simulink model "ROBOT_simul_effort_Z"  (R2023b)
settings: Solver=VariableStepAuto  StartTime=0.0  StopTime=5  RelTol=1e-3
undefined symbols (not defined in the file): deg, kg, m, manette1_Defaut_sldprt, manette2_Defaut_sldprt, mm, N, rad, s, STL, X, Y, Z
libraries: sm_lib x463, fl_lib x45, nesl_utility x27, simulink x2
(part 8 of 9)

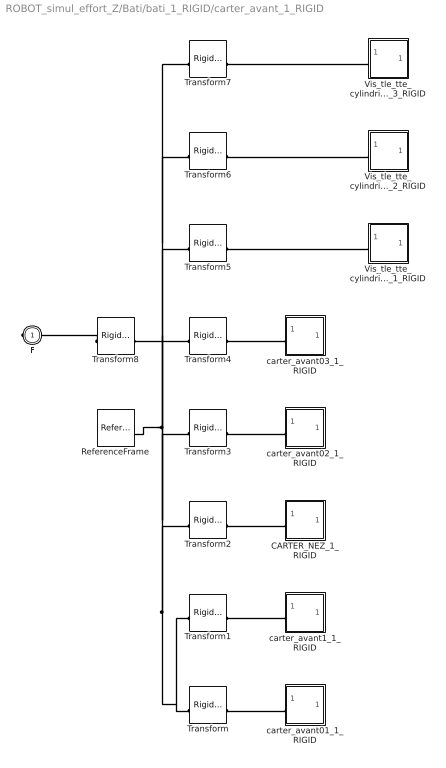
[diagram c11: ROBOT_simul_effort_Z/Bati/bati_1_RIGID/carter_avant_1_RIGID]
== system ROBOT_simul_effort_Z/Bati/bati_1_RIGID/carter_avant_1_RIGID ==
  CARTER_NEZ_1_RIGID : Subsystem
  ReferenceFrame : sm_lib/Frames and Transforms/Reference Frame
  Transform : sm_lib/Frames and Transforms/Rigid Transform  TranslationMethod=Cartesian  TranslationStandardOffset=0  TranslationStandardOffsetUnits=mm  TranslationStandardAxis=+Z  TranslationCartesianOffset=[-17.102622676542445 -113.90982355031112 -1.7985612998927536e-11]  TranslationCartesianOffsetUnits=mm  TranslationROffset=0  TranslationROffsetUnits=m  TranslationZOffset=0  TranslationZOffsetUnits=m  TranslationThetaOffset=0  TranslationThetaOffsetUnits=deg  RotationMethod=None  RotationAngleUnits=deg  RotationStandardAxis=+Z  RotationAngle=0  RotationArbitraryAxis=[0 0 1]  FollAlignAxisA=+X  BaseAlignAxisA=+Y  FollAlignAxisB=+Y  BaseAlignAxisB=+Z  RotationSequenceAxes=FollowerAxes  RotationSequence=XYX  RotationSequenceAngles=[0 0 0]  RotationSequenceAnglesUnits=deg  RotationMatrix=[1 0 0; 0 1 0; 0 0 1]  Quaternion=[1 0 0 0]
  Transform1 : sm_lib/Frames and Transforms/Rigid Transform  TranslationMethod=Cartesian  TranslationStandardOffset=0  TranslationStandardOffsetUnits=mm  TranslationStandardAxis=+Z  TranslationCartesianOffset=[-17.102622676541863 -113.90982355031173 -1.7985612998927536e-11]  TranslationCartesianOffsetUnits=mm  TranslationROffset=0  TranslationROffsetUnits=m  TranslationZOffset=0  TranslationZOffsetUnits=m  TranslationThetaOffset=0  TranslationThetaOffsetUnits=deg  RotationMethod=None  RotationAngleUnits=deg  RotationStandardAxis=+Z  RotationAngle=0  RotationArbitraryAxis=[0 0 1]  FollAlignAxisA=+X  BaseAlignAxisA=+Y  FollAlignAxisB=+Y  BaseAlignAxisB=+Z  RotationSequenceAxes=FollowerAxes  RotationSequence=XYX  RotationSequenceAngles=[0 0 0]  RotationSequenceAnglesUnits=deg  RotationMatrix=[1 0 0; 0 1 0; 0 0 1]  Quaternion=[1 0 0 0]
  Transform2 : sm_lib/Frames and Transforms/Rigid Transform  TranslationMethod=None  TranslationStandardOffset=0  TranslationStandardOffsetUnits=m  TranslationStandardAxis=+Z  TranslationCartesianOffset=[0 0 0]  TranslationCartesianOffsetUnits=m  TranslationROffset=0  TranslationROffsetUnits=m  TranslationZOffset=0  TranslationZOffsetUnits=m  TranslationThetaOffset=0  TranslationThetaOffsetUnits=deg  RotationMethod=ArbitraryAxis  RotationAngleUnits=rad  RotationStandardAxis=+Z  RotationAngle=3.1415926535897931  RotationArbitraryAxis=[0 0.70710678118654746 0.70710678118654757]  FollAlignAxisA=+X  BaseAlignAxisA=+Y  FollAlignAxisB=+Y  BaseAlignAxisB=+Z  RotationSequenceAxes=FollowerAxes  RotationSequence=XYX  RotationSequenceAngles=[0 0 0]  RotationSequenceAnglesUnits=deg  RotationMatrix=[1 0 0; 0 1 0; 0 0 1]  Quaternion=[1 0 0 0]
  Transform3 : sm_lib/Frames and Transforms/Rigid Transform  TranslationMethod=Cartesian  TranslationStandardOffset=0  TranslationStandardOffsetUnits=mm  TranslationStandardAxis=+Z  TranslationCartesianOffset=[82.706805109614251 58.965176449688634 -1.7985612998927536e-11]  TranslationCartesianOffsetUnits=mm  TranslationROffset=0  TranslationROffsetUnits=m  TranslationZOffset=0  TranslationZOffsetUnits=m  TranslationThetaOffset=0  TranslationThetaOffsetUnits=deg  RotationMethod=ArbitraryAxis  RotationAngleUnits=rad  RotationStandardAxis=+Z  RotationAngle=2.094395102393193  RotationArbitraryAxis=[0 0 1]  FollAlignAxisA=+X  BaseAlignAxisA=+Y  FollAlignAxisB=+Y  BaseAlignAxisB=+Z  RotationSequenceAxes=FollowerAxes  RotationSequence=XYX  RotationSequenceAngles=[0 0 0]  RotationSequenceAnglesUnits=deg  RotationMatrix=[1 0 0; 0 1 0; 0 0 1]  Quaternion=[1 0 0 0]
  Transform4 : sm_lib/Frames and Transforms/Rigid Transform  TranslationMethod=Cartesian  TranslationStandardOffset=0  TranslationStandardOffsetUnits=mm  TranslationStandardAxis=+Z  TranslationCartesianOffset=[-116.91205046269873 58.965176449689402 -1.7985612998927536e-11]  TranslationCartesianOffsetUnits=mm  TranslationROffset=0  TranslationROffsetUnits=m  TranslationZOffset=0  TranslationZOffsetUnits=m  TranslationThetaOffset=0  TranslationThetaOffsetUnits=deg  RotationMethod=ArbitraryAxis  RotationAngleUnits=rad  RotationStandardAxis=+Z  RotationAngle=2.0943951023932006  RotationArbitraryAxis=[-0 -0 -1]  FollAlignAxisA=+X  BaseAlignAxisA=+Y  FollAlignAxisB=+Y  BaseAlignAxisB=+Z  RotationSequenceAxes=FollowerAxes  RotationSequence=XYX  RotationSequenceAngles=[0 0 0]  RotationSequenceAnglesUnits=deg  RotationMatrix=[1 0 0; 0 1 0; 0 0 1]  Quaternion=[1 0 0 0]
  Transform5 : sm_lib/Frames and Transforms/Rigid Transform  TranslationMethod=Cartesian  TranslationStandardOffset=0  TranslationStandardOffsetUnits=mm  TranslationStandardAxis=+Z  TranslationCartesianOffset=[-32.01022121330513 -41.991412127562512 96.999999999981995]  TranslationCartesianOffsetUnits=mm  TranslationROffset=0  TranslationROffsetUnits=m  TranslationZOffset=0  TranslationZOffsetUnits=m  TranslationThetaOffset=0  TranslationThetaOffsetUnits=deg  RotationMethod=ArbitraryAxis  RotationAngleUnits=rad  RotationStandardAxis=+Z  RotationAngle=1.5707963267948968  RotationArbitraryAxis=[0 1 0]  FollAlignAxisA=+X  BaseAlignAxisA=+Y  FollAlignAxisB=+Y  BaseAlignAxisB=+Z  RotationSequenceAxes=FollowerAxes  RotationSequence=XYX  RotationSequenceAngles=[0 0 0]  RotationSequenceAnglesUnits=deg  RotationMatrix=[1 0 0; 0 1 0; 0 0 1]  Quaternion=[1 0 0 0]
  Transform6 : sm_lib/Frames and Transforms/Rigid Transform  TranslationMethod=Cartesian  TranslationStandardOffset=0  TranslationStandardOffsetUnits=mm  TranslationStandardAxis=+Z  TranslationCartesianOffset=[-47.17507990239649 35.916329780570692 96.999999999981995]  TranslationCartesianOffsetUnits=mm  TranslationROffset=0  TranslationROffsetUnits=m  TranslationZOffset=0  TranslationZOffsetUnits=m  TranslationThetaOffset=0  TranslationThetaOffsetUnits=deg  RotationMethod=ArbitraryAxis  RotationAngleUnits=rad  RotationStandardAxis=+Z  RotationAngle=1.5707963267948968  RotationArbitraryAxis=[0 1 0]  FollAlignAxisA=+X  BaseAlignAxisA=+Y  FollAlignAxisB=+Y  BaseAlignAxisB=+Z  RotationSequenceAxes=FollowerAxes  RotationSequence=XYX  RotationSequenceAngles=[0 0 0]  RotationSequenceAnglesUnits=deg  RotationMatrix=[1 0 0; 0 1 0; 0 0 1]  Quaternion=[1 0 0 0]
  Transform7 : sm_lib/Frames and Transforms/Rigid Transform  TranslationMethod=Cartesian  TranslationStandardOffset=0  TranslationStandardOffsetUnits=mm  TranslationStandardAxis=+Z  TranslationCartesianOffset=[27.877433086074202 10.09561169605827 96.999999999981995]  TranslationCartesianOffsetUnits=mm  TranslationROffset=0  TranslationROffsetUnits=m  TranslationZOffset=0  TranslationZOffsetUnits=m  TranslationThetaOffset=0  TranslationThetaOffsetUnits=deg  RotationMethod=ArbitraryAxis  RotationAngleUnits=rad  RotationStandardAxis=+Z  RotationAngle=1.5707963267948968  RotationArbitraryAxis=[0 1 0]  FollAlignAxisA=+X  BaseAlignAxisA=+Y  FollAlignAxisB=+Y  BaseAlignAxisB=+Z  RotationSequenceAxes=FollowerAxes  RotationSequence=XYX  RotationSequenceAngles=[0 0 0]  RotationSequenceAnglesUnits=deg  RotationMatrix=[1 0 0; 0 1 0; 0 0 1]  Quaternion=[1 0 0 0]
  Transform8 : sm_lib/Frames and Transforms/Rigid Transform  TranslationMethod=Cartesian  TranslationStandardOffset=0  TranslationStandardOffsetUnits=mm  TranslationStandardAxis=+Z  TranslationCartesianOffset=[17.102622676542548 113.90982355031109 24.00000000001798]  TranslationCartesianOffsetUnits=mm  TranslationROffset=0  TranslationROffsetUnits=m  TranslationZOffset=0  TranslationZOffsetUnits=m  TranslationThetaOffset=0  TranslationThetaOffsetUnits=deg  RotationMethod=None  RotationAngleUnits=deg  RotationStandardAxis=+Z  RotationAngle=0  RotationArbitraryAxis=[0 0 1]  FollAlignAxisA=+X  BaseAlignAxisA=+Y  FollAlignAxisB=+Y  BaseAlignAxisB=+Z  RotationSequenceAxes=FollowerAxes  RotationSequence=XYX  RotationSequenceAngles=[0 0 0]  RotationSequenceAnglesUnits=deg  RotationMatrix=[1 0 0; 0 1 0; 0 0 1]  Quaternion=[1 0 0 0]
  Vis_tle_tte_cylindrique_cruciforme_H_29x13_C_1_RIGID : Subsystem
  Vis_tle_tte_cylindrique_cruciforme_H_29x13_C_2_RIGID : Subsystem
  Vis_tle_tte_cylindrique_cruciforme_H_29x13_C_3_RIGID : Subsystem
  carter_avant01_1_RIGID : Subsystem
  carter_avant02_1_RIGID : Subsystem
  carter_avant03_1_RIGID : Subsystem
  carter_avant1_1_RIGID : Subsystem
  F : PMIOPort  Side=Right
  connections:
  Transform/RConn1 -- carter_avant01_1_RIGID/LConn1
  Transform1/RConn1 -- carter_avant1_1_RIGID/LConn1
  CARTER_NEZ_1_RIGID/LConn1 -- Transform2/RConn1
  Transform3/RConn1 -- carter_avant02_1_RIGID/LConn1
  Transform4/RConn1 -- carter_avant03_1_RIGID/LConn1
  Transform5/RConn1 -- Vis_tle_tte_cylindrique_cruciforme_H_29x13_C_1_RIGID/LConn1
  Transform6/RConn1 -- Vis_tle_tte_cylindrique_cruciforme_H_29x13_C_2_RIGID/LConn1
  Transform7/RConn1 -- Vis_tle_tte_cylindrique_cruciforme_H_29x13_C_3_RIGID/LConn1
  Transform/LConn1 -- Transform6/LConn1 -- Transform7/LConn1 -- Transform5/LConn1 -- Transform4/LConn1 -- ReferenceFrame/RConn1 -- Transform8/RConn1 -- Transform3/LConn1 -- Transform2/LConn1 -- Transform1/LConn1
  Transform8/LConn1 -- F/RConn1

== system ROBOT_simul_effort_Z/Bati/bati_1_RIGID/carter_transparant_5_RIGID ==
  ReferenceFrame : sm_lib/Frames and Transforms/Reference Frame
  Transform : sm_lib/Frames and Transforms/Rigid Transform  TranslationMethod=Cartesian  TranslationStandardOffset=0  TranslationStandardOffsetUnits=mm  TranslationStandardAxis=+Z  TranslationCartesianOffset=[-114.07592590479371 112.90132228455712 35.212494571905935]  TranslationCartesianOffsetUnits=mm  TranslationROffset=0  TranslationROffsetUnits=m  TranslationZOffset=0  TranslationZOffsetUnits=m  TranslationThetaOffset=0  TranslationThetaOffsetUnits=deg  RotationMethod=ArbitraryAxis  RotationAngleUnits=rad  RotationStandardAxis=+Z  RotationAngle=2.0943951023932001  RotationArbitraryAxis=[-0 -0 -1]  FollAlignAxisA=+X  BaseAlignAxisA=+Y  FollAlignAxisB=+Y  BaseAlignAxisB=+Z  RotationSequenceAxes=FollowerAxes  RotationSequence=XYX  RotationSequenceAngles=[0 0 0]  RotationSequenceAnglesUnits=deg  RotationMatrix=[1 0 0; 0 1 0; 0 0 1]  Quaternion=[1 0 0 0]
  Transform1 : sm_lib/Frames and Transforms/Rigid Transform  TranslationMethod=Cartesian  TranslationStandardOffset=0  TranslationStandardOffsetUnits=mm  TranslationStandardAxis=+Z  TranslationCartesianOffset=[-14.266498118637394 -59.973677715443351 35.212494571905921]  TranslationCartesianOffsetUnits=mm  TranslationROffset=0  TranslationROffsetUnits=m  TranslationZOffset=0  TranslationZOffsetUnits=m  TranslationThetaOffset=0  TranslationThetaOffsetUnits=deg  RotationMethod=None  RotationAngleUnits=deg  RotationStandardAxis=+Z  RotationAngle=0  RotationArbitraryAxis=[0 0 1]  FollAlignAxisA=+X  BaseAlignAxisA=+Y  FollAlignAxisB=+Y  BaseAlignAxisB=+Z  RotationSequenceAxes=FollowerAxes  RotationSequence=XYX  RotationSequenceAngles=[0 0 0]  RotationSequenceAnglesUnits=deg  RotationMatrix=[1 0 0; 0 1 0; 0 0 1]  Quaternion=[1 0 0 0]
  Transform2 : sm_lib/Frames and Transforms/Rigid Transform  TranslationMethod=Cartesian  TranslationStandardOffset=0  TranslationStandardOffsetUnits=mm  TranslationStandardAxis=+Z  TranslationCartesianOffset=[85.542929667519687 112.90132228455593 35.212494571905921]  TranslationCartesianOffsetUnits=mm  TranslationROffset=0  TranslationROffsetUnits=m  TranslationZOffset=0  TranslationZOffsetUnits=m  TranslationThetaOffset=0  TranslationThetaOffsetUnits=deg  RotationMethod=ArbitraryAxis  RotationAngleUnits=rad  RotationStandardAxis=+Z  RotationAngle=2.0943951023931877  RotationArbitraryAxis=[0 0 1]  FollAlignAxisA=+X  BaseAlignAxisA=+Y  FollAlignAxisB=+Y  BaseAlignAxisB=+Z  RotationSequenceAxes=FollowerAxes  RotationSequence=XYX  RotationSequenceAngles=[0 0 0]  RotationSequenceAnglesUnits=deg  RotationMatrix=[1 0 0; 0 1 0; 0 0 1]  Quaternion=[1 0 0 0]
  Transform3 : sm_lib/Frames and Transforms/Rigid Transform  TranslationMethod=Cartesian  TranslationStandardOffset=0  TranslationStandardOffsetUnits=mm  TranslationStandardAxis=+Z  TranslationCartesianOffset=[12.872893350874152 59.632616111037024 -35.212494571905921]  TranslationCartesianOffsetUnits=mm  TranslationROffset=0  TranslationROffsetUnits=m  TranslationZOffset=0  TranslationZOffsetUnits=m  TranslationThetaOffset=0  TranslationThetaOffsetUnits=deg  RotationMethod=ArbitraryAxis  RotationAngleUnits=rad  RotationStandardAxis=+Z  RotationAngle=0.025132741228718395  RotationArbitraryAxis=[0 0 -1]  FollAlignAxisA=+X  BaseAlignAxisA=+Y  FollAlignAxisB=+Y  BaseAlignAxisB=+Z  RotationSequenceAxes=FollowerAxes  RotationSequence=XYX  RotationSequenceAngles=[0 0 0]  RotationSequenceAnglesUnits=deg  RotationMatrix=[1 0 0; 0 1 0; 0 0 1]  Quaternion=[1 0 0 0]
  carter_transparent2_1_RIGID : Subsystem
  carter_transparent_1_RIGID : Subsystem
  carter_transparent_modif_matlab_1_RIGID : Subsystem
  F : PMIOPort  Side=Right
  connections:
  Transform/RConn1 -- carter_transparent_1_RIGID/LConn1
  Transform1/RConn1 -- carter_transparent2_1_RIGID/LConn1
  Transform2/RConn1 -- carter_transparent_modif_matlab_1_RIGID/LConn1
  Transform/LConn1 -- Transform1/LConn1 -- Transform2/LConn1 -- ReferenceFrame/RConn1 -- Transform3/RConn1
  Transform3/LConn1 -- F/RConn1

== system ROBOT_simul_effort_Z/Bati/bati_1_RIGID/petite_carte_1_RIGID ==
  ReferenceFrame : sm_lib/Frames and Transforms/Reference Frame
  Solid : sm_lib/Body Elements/File Solid  ExtGeomFileName=\STL\petite carte_Defaut_sldprt.STL  UnitType=Custom  ExtGeomFileUnits=mm  StepReaderType=HEX  ExportConvexHullGeometry=off  InertiaType=Custom  Mass=0.00048082183649251445  MassUnits=kg  CenterOfMass=[19.91458998704724 1.4286045215267169 0.6668228749994265]  CenterOfMassUnits=mm  MomentsOfInertia=[0.0075326471062909569 0.048633515547401453 0.053492974016950315]  MomentsOfInertiaUnits=kg*mm^2  ProductsOfInertia=[9.9546833043094831e-05 0.0011485008863759011 0.0086575785704640102]  ProductsOfInertiaUnits=kg*mm^2  BasedOnType=Density  Density=1000  DensityUnits=kg/(m^3)  DoExposeReferenceFrame=on  SerializedFrames=<Frames/>  GraphicType=FromGeometry  MarkerShape=Sphere  MarkerSize=10  MarkerSizeUnits=m  GraphicVisPropType=SimpleVisualProperties  GraphicDiffuseColor=[0 0.50196078431372548 0]  GraphicSpecularColor=[0.5 0.5 0.5 1.0]  GraphicAmbientColor=[0.15 0.15 0.15 1.0]  GraphicEmissiveColor=[0.0 0.0 0.0 1.0]  GraphicShininess=75  GraphicOpacity=1
  F : PMIOPort  Side=Left
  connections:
  Solid/RConn1 -- ReferenceFrame/RConn1 -- F/RConn1

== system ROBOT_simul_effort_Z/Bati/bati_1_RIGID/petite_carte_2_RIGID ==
  ReferenceFrame : sm_lib/Frames and Transforms/Reference Frame
  Solid : sm_lib/Body Elements/File Solid  ExtGeomFileName=\STL\petite carte_Defaut_sldprt.STL  UnitType=Custom  ExtGeomFileUnits=mm  StepReaderType=HEX  ExportConvexHullGeometry=off  InertiaType=Custom  Mass=0.00048082183649251445  MassUnits=kg  CenterOfMass=[19.91458998704724 1.4286045215267169 0.6668228749994265]  CenterOfMassUnits=mm  MomentsOfInertia=[0.0075326471062909569 0.048633515547401453 0.053492974016950315]  MomentsOfInertiaUnits=kg*mm^2  ProductsOfInertia=[9.9546833043094831e-05 0.0011485008863759011 0.0086575785704640102]  ProductsOfInertiaUnits=kg*mm^2  BasedOnType=Density  Density=1000  DensityUnits=kg/(m^3)  DoExposeReferenceFrame=on  SerializedFrames=<Frames/>  GraphicType=FromGeometry  MarkerShape=Sphere  MarkerSize=10  MarkerSizeUnits=m  GraphicVisPropType=SimpleVisualProperties  GraphicDiffuseColor=[0 0.50196078431372548 0]  GraphicSpecularColor=[0.5 0.5 0.5 1.0]  GraphicAmbientColor=[0.15 0.15 0.15 1.0]  GraphicEmissiveColor=[0.0 0.0 0.0 1.0]  GraphicShininess=75  GraphicOpacity=1
  F : PMIOPort  Side=Left
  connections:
  Solid/RConn1 -- ReferenceFrame/RConn1 -- F/RConn1

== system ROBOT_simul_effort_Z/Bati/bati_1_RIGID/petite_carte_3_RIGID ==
  ReferenceFrame : sm_lib/Frames and Transforms/Reference Frame
  Solid : sm_lib/Body Elements/File Solid  ExtGeomFileName=\STL\petite carte_Defaut_sldprt.STL  UnitType=Custom  ExtGeomFileUnits=mm  StepReaderType=HEX  ExportConvexHullGeometry=off  InertiaType=Custom  Mass=0.00048082183649251445  MassUnits=kg  CenterOfMass=[19.91458998704724 1.4286045215267169 0.6668228749994265]  CenterOfMassUnits=mm  MomentsOfInertia=[0.0075326471062909569 0.048633515547401453 0.053492974016950315]  MomentsOfInertiaUnits=kg*mm^2  ProductsOfInertia=[9.9546833043094831e-05 0.0011485008863759011 0.0086575785704640102]  ProductsOfInertiaUnits=kg*mm^2  BasedOnType=Density  Density=1000  DensityUnits=kg/(m^3)  DoExposeReferenceFrame=on  SerializedFrames=<Frames/>  GraphicType=FromGeometry  MarkerShape=Sphere  MarkerSize=10  MarkerSizeUnits=m  GraphicVisPropType=SimpleVisualProperties  GraphicDiffuseColor=[0 0.50196078431372548 0]  GraphicSpecularColor=[0.5 0.5 0.5 1.0]  GraphicAmbientColor=[0.15 0.15 0.15 1.0]  GraphicEmissiveColor=[0.0 0.0 0.0 1.0]  GraphicShininess=75  GraphicOpacity=1
  F : PMIOPort  Side=Left
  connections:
  Solid/RConn1 -- ReferenceFrame/RConn1 -- F/RConn1

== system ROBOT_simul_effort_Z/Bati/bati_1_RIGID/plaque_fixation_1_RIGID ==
  ReferenceFrame : sm_lib/Frames and Transforms/Reference Frame
  Solid : sm_lib/Body Elements/File Solid  ExtGeomFileName=\STL\plaque fixation_Defaut_sldprt.STL  UnitType=Custom  ExtGeomFileUnits=mm  StepReaderType=HEX  ExportConvexHullGeometry=off  InertiaType=Custom  Mass=0.13619587212093154  MassUnits=kg  CenterOfMass=[0 57.644814512190067 6.7752904956014124]  CenterOfMassUnits=mm  MomentsOfInertia=[230.56748251711528 59.503021506275417 273.91192419339654]  MomentsOfInertiaUnits=kg*mm^2  ProductsOfInertia=[16.91481201365259 0 0]  ProductsOfInertiaUnits=kg*mm^2  BasedOnType=Density  Density=1000  DensityUnits=kg/(m^3)  DoExposeReferenceFrame=on  SerializedFrames=<Frames/>  GraphicType=FromGeometry  MarkerShape=Sphere  MarkerSize=10  MarkerSizeUnits=m  GraphicVisPropType=SimpleVisualProperties  GraphicDiffuseColor=[0.6470588235294118 0.61960784313725492 0.58823529411764708]  GraphicSpecularColor=[0.5 0.5 0.5 1.0]  GraphicAmbientColor=[0.15 0.15 0.15 1.0]  GraphicEmissiveColor=[0.0 0.0 0.0 1.0]  GraphicShininess=75  GraphicOpacity=1
  F : PMIOPort  Side=Left
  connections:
  Solid/RConn1 -- ReferenceFrame/RConn1 -- F/RConn1

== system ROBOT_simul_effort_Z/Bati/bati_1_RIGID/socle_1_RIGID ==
  ReferenceFrame : sm_lib/Frames and Transforms/Reference Frame
  Solid : sm_lib/Body Elements/File Solid  ExtGeomFileName=\STL\socle_Defaut_sldprt.STL  UnitType=Custom  ExtGeomFileUnits=mm  StepReaderType=HEX  ExportConvexHullGeometry=off  InertiaType=Custom  Mass=0.22494978957848721  MassUnits=kg  CenterOfMass=[-0.04792533570938888 16.018647482078187 6.7264124950212594]  CenterOfMassUnits=mm  MomentsOfInertia=[992.11143480501664 1618.7630611955949 2601.3810500563377]  MomentsOfInertiaUnits=kg*mm^2  ProductsOfInertia=[-5.1990662975402211 -0.041150083489637494 0.38689094335060764]  ProductsOfInertiaUnits=kg*mm^2  BasedOnType=Density  Density=1000  DensityUnits=kg/(m^3)  DoExposeReferenceFrame=on  SerializedFrames=<Frames/>  GraphicType=FromGeometry  MarkerShape=Sphere  MarkerSize=10  MarkerSizeUnits=m  GraphicVisPropType=SimpleVisualProperties  GraphicDiffuseColor=[0.792156862745098 0.81960784313725488 0.93333333333333335]  GraphicSpecularColor=[0.5 0.5 0.5 1.0]  GraphicAmbientColor=[0.15 0.15 0.15 1.0]  GraphicEmissiveColor=[0.0 0.0 0.0 1.0]  GraphicShininess=75  GraphicOpacity=1
  F : PMIOPort  Side=Left
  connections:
  Solid/RConn1 -- ReferenceFrame/RConn1 -- F/RConn1

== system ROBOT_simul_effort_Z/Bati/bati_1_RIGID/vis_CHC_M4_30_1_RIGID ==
  ReferenceFrame : sm_lib/Frames and Transforms/Reference Frame
  Solid : sm_lib/Body Elements/File Solid  ExtGeomFileName=\STL\vis CHC M4-30_Defaut_sldprt.STL  UnitType=Custom  ExtGeomFileUnits=mm  StepReaderType=HEX  ExportConvexHullGeometry=off  InertiaType=Custom  Mass=0.00050829612748328964  MassUnits=kg  CenterOfMass=[0 0 19.413574172112984]  CenterOfMassUnits=mm  MomentsOfInertia=[0.056747582392929367 0.056747582392929367 0.0016443905083794684]  MomentsOfInertiaUnits=kg*mm^2  ProductsOfInertia=[0 0 0]  ProductsOfInertiaUnits=kg*mm^2  BasedOnType=Density  Density=1000  DensityUnits=kg/(m^3)  DoExposeReferenceFrame=on  SerializedFrames=<Frames/>  GraphicType=FromGeometry  MarkerShape=Sphere  MarkerSize=10  MarkerSizeUnits=m  GraphicVisPropType=SimpleVisualProperties  GraphicDiffuseColor=[0.75294117647058822 0.75294117647058822 0.75294117647058822]  GraphicSpecularColor=[0.5 0.5 0.5 1.0]  GraphicAmbientColor=[0.15 0.15 0.15 1.0]  GraphicEmissiveColor=[0.0 0.0 0.0 1.0]  GraphicShininess=75  GraphicOpacity=1
  F : PMIOPort  Side=Left
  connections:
  Solid/RConn1 -- ReferenceFrame/RConn1 -- F/RConn1

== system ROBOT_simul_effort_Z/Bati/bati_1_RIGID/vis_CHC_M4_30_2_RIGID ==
  ReferenceFrame : sm_lib/Frames and Transforms/Reference Frame
  Solid : sm_lib/Body Elements/File Solid  ExtGeomFileName=\STL\vis CHC M4-30_Defaut_sldprt.STL  UnitType=Custom  ExtGeomFileUnits=mm  StepReaderType=HEX  ExportConvexHullGeometry=off  InertiaType=Custom  Mass=0.00050829612748328964  MassUnits=kg  CenterOfMass=[0 0 19.413574172112984]  CenterOfMassUnits=mm  MomentsOfInertia=[0.056747582392929367 0.056747582392929367 0.0016443905083794684]  MomentsOfInertiaUnits=kg*mm^2  ProductsOfInertia=[0 0 0]  ProductsOfInertiaUnits=kg*mm^2  BasedOnType=Density  Density=1000  DensityUnits=kg/(m^3)  DoExposeReferenceFrame=on  SerializedFrames=<Frames/>  GraphicType=FromGeometry  MarkerShape=Sphere  MarkerSize=10  MarkerSizeUnits=m  GraphicVisPropType=SimpleVisualProperties  GraphicDiffuseColor=[0.75294117647058822 0.75294117647058822 0.75294117647058822]  GraphicSpecularColor=[0.5 0.5 0.5 1.0]  GraphicAmbientColor=[0.15 0.15 0.15 1.0]  GraphicEmissiveColor=[0.0 0.0 0.0 1.0]  GraphicShininess=75  GraphicOpacity=1
  F : PMIOPort  Side=Left
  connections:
  Solid/RConn1 -- ReferenceFrame/RConn1 -- F/RConn1

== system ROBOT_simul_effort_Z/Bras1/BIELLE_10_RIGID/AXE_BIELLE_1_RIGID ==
  ReferenceFrame : sm_lib/Frames and Transforms/Reference Frame
  Solid : sm_lib/Body Elements/File Solid  ExtGeomFileName=\STL\AXE BIELLE_Defaut_sldprt.STL  UnitType=Custom  ExtGeomFileUnits=mm  StepReaderType=HEX  ExportConvexHullGeometry=off  InertiaType=Custom  Mass=0.0008880235381781051  MassUnits=kg  CenterOfMass=[0 0 0]  CenterOfMassUnits=mm  MomentsOfInertia=[0.018768660222737772 0.018768660222737772 0.0009874025874388381]  MomentsOfInertiaUnits=kg*mm^2  ProductsOfInertia=[0 0 0]  ProductsOfInertiaUnits=kg*mm^2  BasedOnType=Density  Density=1000  DensityUnits=kg/(m^3)  DoExposeReferenceFrame=on  SerializedFrames=<Frames/>  GraphicType=FromGeometry  MarkerShape=Sphere  MarkerSize=10  MarkerSizeUnits=m  GraphicVisPropType=SimpleVisualProperties  GraphicDiffuseColor=[1 0.94901960784313721 0.90980392156862744]  GraphicSpecularColor=[0.5 0.5 0.5 1.0]  GraphicAmbientColor=[0.15 0.15 0.15 1.0]  GraphicEmissiveColor=[0.0 0.0 0.0 1.0]  GraphicShininess=75  GraphicOpacity=1
  F : PMIOPort  Side=Left
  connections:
  Solid/RConn1 -- ReferenceFrame/RConn1 -- F/RConn1

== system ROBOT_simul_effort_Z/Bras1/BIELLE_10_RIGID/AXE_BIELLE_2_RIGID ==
  ReferenceFrame : sm_lib/Frames and Transforms/Reference Frame
  Solid : sm_lib/Body Elements/File Solid  ExtGeomFileName=\STL\AXE BIELLE_Defaut_sldprt.STL  UnitType=Custom  ExtGeomFileUnits=mm  StepReaderType=HEX  ExportConvexHullGeometry=off  InertiaType=Custom  Mass=0.0008880235381781051  MassUnits=kg  CenterOfMass=[0 0 0]  CenterOfMassUnits=mm  MomentsOfInertia=[0.018768660222737772 0.018768660222737772 0.0009874025874388381]  MomentsOfInertiaUnits=kg*mm^2  ProductsOfInertia=[0 0 0]  ProductsOfInertiaUnits=kg*mm^2  BasedOnType=Density  Density=1000  DensityUnits=kg/(m^3)  DoExposeReferenceFrame=on  SerializedFrames=<Frames/>  GraphicType=FromGeometry  MarkerShape=Sphere  MarkerSize=10  MarkerSizeUnits=m  GraphicVisPropType=SimpleVisualProperties  GraphicDiffuseColor=[1 0.94901960784313721 0.90980392156862744]  GraphicSpecularColor=[0.5 0.5 0.5 1.0]  GraphicAmbientColor=[0.15 0.15 0.15 1.0]  GraphicEmissiveColor=[0.0 0.0 0.0 1.0]  GraphicShininess=75  GraphicOpacity=1
  F : PMIOPort  Side=Left
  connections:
  Solid/RConn1 -- ReferenceFrame/RConn1 -- F/RConn1

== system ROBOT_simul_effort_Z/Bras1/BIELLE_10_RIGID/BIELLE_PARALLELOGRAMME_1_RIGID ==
  ReferenceFrame : sm_lib/Frames and Transforms/Reference Frame
  Solid : sm_lib/Body Elements/File Solid  ExtGeomFileName=\STL\BIELLE PARALLELOGRAMME_Defaut_sldprt.STL  UnitType=Custom  ExtGeomFileUnits=mm  StepReaderType=HEX  ExportConvexHullGeometry=off  InertiaType=Custom  Mass=0.0079529027635324764  MassUnits=kg  CenterOfMass=[0 3.1653377955585489 0]  CenterOfMassUnits=mm  MomentsOfInertia=[7.7987017961340088 7.8475939194203406 0.14816857834406802]  MomentsOfInertiaUnits=kg*mm^2  ProductsOfInertia=[0 0 0]  ProductsOfInertiaUnits=kg*mm^2  BasedOnType=Density  Density=1000  DensityUnits=kg/(m^3)  DoExposeReferenceFrame=on  SerializedFrames=<Frames/>  GraphicType=FromGeometry  MarkerShape=Sphere  MarkerSize=10  MarkerSizeUnits=m  GraphicVisPropType=SimpleVisualProperties  GraphicDiffuseColor=[0.6 1.0 1.0]  GraphicSpecularColor=[0.5 0.5 0.5 1.0]  GraphicAmbientColor=[0.15 0.15 0.15 1.0]  GraphicEmissiveColor=[0.0 0.0 0.0 1.0]  GraphicShininess=75  GraphicOpacity=1
  F : PMIOPort  Side=Left
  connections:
  Solid/RConn1 -- ReferenceFrame/RConn1 -- F/RConn1

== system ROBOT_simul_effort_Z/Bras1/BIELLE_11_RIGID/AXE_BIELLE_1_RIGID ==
  ReferenceFrame : sm_lib/Frames and Transforms/Reference Frame
  Solid : sm_lib/Body Elements/File Solid  ExtGeomFileName=\STL\AXE BIELLE_Defaut_sldprt.STL  UnitType=Custom  ExtGeomFileUnits=mm  StepReaderType=HEX  ExportConvexHullGeometry=off  InertiaType=Custom  Mass=0.0008880235381781051  MassUnits=kg  CenterOfMass=[0 0 0]  CenterOfMassUnits=mm  MomentsOfInertia=[0.018768660222737772 0.018768660222737772 0.0009874025874388381]  MomentsOfInertiaUnits=kg*mm^2  ProductsOfInertia=[0 0 0]  ProductsOfInertiaUnits=kg*mm^2  BasedOnType=Density  Density=1000  DensityUnits=kg/(m^3)  DoExposeReferenceFrame=on  SerializedFrames=<Frames/>  GraphicType=FromGeometry  MarkerShape=Sphere  MarkerSize=10  MarkerSizeUnits=m  GraphicVisPropType=SimpleVisualProperties  GraphicDiffuseColor=[1 0.94901960784313721 0.90980392156862744]  GraphicSpecularColor=[0.5 0.5 0.5 1.0]  GraphicAmbientColor=[0.15 0.15 0.15 1.0]  GraphicEmissiveColor=[0.0 0.0 0.0 1.0]  GraphicShininess=75  GraphicOpacity=1
  F : PMIOPort  Side=Left
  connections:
  Solid/RConn1 -- ReferenceFrame/RConn1 -- F/RConn1

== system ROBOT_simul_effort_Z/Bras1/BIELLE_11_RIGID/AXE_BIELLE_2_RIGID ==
  ReferenceFrame : sm_lib/Frames and Transforms/Reference Frame
  Solid : sm_lib/Body Elements/File Solid  ExtGeomFileName=\STL\AXE BIELLE_Defaut_sldprt.STL  UnitType=Custom  ExtGeomFileUnits=mm  StepReaderType=HEX  ExportConvexHullGeometry=off  InertiaType=Custom  Mass=0.0008880235381781051  MassUnits=kg  CenterOfMass=[0 0 0]  CenterOfMassUnits=mm  MomentsOfInertia=[0.018768660222737772 0.018768660222737772 0.0009874025874388381]  MomentsOfInertiaUnits=kg*mm^2  ProductsOfInertia=[0 0 0]  ProductsOfInertiaUnits=kg*mm^2  BasedOnType=Density  Density=1000  DensityUnits=kg/(m^3)  DoExposeReferenceFrame=on  SerializedFrames=<Frames/>  GraphicType=FromGeometry  MarkerShape=Sphere  MarkerSize=10  MarkerSizeUnits=m  GraphicVisPropType=SimpleVisualProperties  GraphicDiffuseColor=[1 0.94901960784313721 0.90980392156862744]  GraphicSpecularColor=[0.5 0.5 0.5 1.0]  GraphicAmbientColor=[0.15 0.15 0.15 1.0]  GraphicEmissiveColor=[0.0 0.0 0.0 1.0]  GraphicShininess=75  GraphicOpacity=1
  F : PMIOPort  Side=Left
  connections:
  Solid/RConn1 -- ReferenceFrame/RConn1 -- F/RConn1

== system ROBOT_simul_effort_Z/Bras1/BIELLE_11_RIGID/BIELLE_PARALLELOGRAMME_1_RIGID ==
  ReferenceFrame : sm_lib/Frames and Transforms/Reference Frame
  Solid : sm_lib/Body Elements/File Solid  ExtGeomFileName=\STL\BIELLE PARALLELOGRAMME_Defaut_sldprt.STL  UnitType=Custom  ExtGeomFileUnits=mm  StepReaderType=HEX  ExportConvexHullGeometry=off  InertiaType=Custom  Mass=0.0079529027635324764  MassUnits=kg  CenterOfMass=[0 3.1653377955585489 0]  CenterOfMassUnits=mm  MomentsOfInertia=[7.7987017961340088 7.8475939194203406 0.14816857834406802]  MomentsOfInertiaUnits=kg*mm^2  ProductsOfInertia=[0 0 0]  ProductsOfInertiaUnits=kg*mm^2  BasedOnType=Density  Density=1000  DensityUnits=kg/(m^3)  DoExposeReferenceFrame=on  SerializedFrames=<Frames/>  GraphicType=FromGeometry  MarkerShape=Sphere  MarkerSize=10  MarkerSizeUnits=m  GraphicVisPropType=SimpleVisualProperties  GraphicDiffuseColor=[0.6 1.0 1.0]  GraphicSpecularColor=[0.5 0.5 0.5 1.0]  GraphicAmbientColor=[0.15 0.15 0.15 1.0]  GraphicEmissiveColor=[0.0 0.0 0.0 1.0]  GraphicShininess=75  GraphicOpacity=1
  F : PMIOPort  Side=Left
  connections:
  Solid/RConn1 -- ReferenceFrame/RConn1 -- F/RConn1

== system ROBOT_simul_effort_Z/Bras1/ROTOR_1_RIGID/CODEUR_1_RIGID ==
  ReferenceFrame : sm_lib/Frames and Transforms/Reference Frame
  Solid : sm_lib/Body Elements/File Solid  ExtGeomFileName=\STL\CODEUR_Defaut_sldprt.STL  UnitType=Custom  ExtGeomFileUnits=mm  StepReaderType=HEX  ExportConvexHullGeometry=off  InertiaType=Custom  Mass=0.0064318274490095598  MassUnits=kg  CenterOfMass=[0 6.0527709306807029 -0.1964144966449296]  CenterOfMassUnits=mm  MomentsOfInertia=[0.92812714377460337 1.2443807481520079 0.93469179577802664]  MomentsOfInertiaUnits=kg*mm^2  ProductsOfInertia=[0.0063987198741970201 0 0]  ProductsOfInertiaUnits=kg*mm^2  BasedOnType=Density  Density=1000  DensityUnits=kg/(m^3)  DoExposeReferenceFrame=on  SerializedFrames=<Frames/>  GraphicType=FromGeometry  MarkerShape=Sphere  MarkerSize=10  MarkerSizeUnits=m  GraphicVisPropType=SimpleVisualProperties  GraphicDiffuseColor=[0.2 1.0 0.0]  GraphicSpecularColor=[0.5 0.5 0.5 1.0]  GraphicAmbientColor=[0.15 0.15 0.15 1.0]  GraphicEmissiveColor=[0.0 0.0 0.0 1.0]  GraphicShininess=75  GraphicOpacity=1
  F : PMIOPort  Side=Left
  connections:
  Solid/RConn1 -- ReferenceFrame/RConn1 -- F/RConn1

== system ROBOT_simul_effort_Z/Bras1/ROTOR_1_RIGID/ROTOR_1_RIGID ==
  ReferenceFrame : sm_lib/Frames and Transforms/Reference Frame
  Solid : sm_lib/Body Elements/File Solid  ExtGeomFileName=\STL\ROTOR_Defaut_sldprt.STL  UnitType=Custom  ExtGeomFileUnits=mm  StepReaderType=HEX  ExportConvexHullGeometry=off  InertiaType=Custom  Mass=0.07643998420030651  MassUnits=kg  CenterOfMass=[0 30.928341108151987 -0.0018262913863015125]  CenterOfMassUnits=mm  MomentsOfInertia=[14.640748377051393 9.6696912582654697 14.640902193857929]  MomentsOfInertiaUnits=kg*mm^2  ProductsOfInertia=[0.0065014820412302417 0 0]  ProductsOfInertiaUnits=kg*mm^2  BasedOnType=Density  Density=1000  DensityUnits=kg/(m^3)  DoExposeReferenceFrame=on  SerializedFrames=<Frames/>  GraphicType=FromGeometry  MarkerShape=Sphere  MarkerSize=10  MarkerSizeUnits=m  GraphicVisPropType=SimpleVisualProperties  GraphicDiffuseColor=[0.53725490196078429 0.34901960784313724 0.33725490196078434]  GraphicSpecularColor=[0.5 0.5 0.5 1.0]  GraphicAmbientColor=[0.15 0.15 0.15 1.0]  GraphicEmissiveColor=[0.0 0.0 0.0 1.0]  GraphicShininess=75  GraphicOpacity=1
  F : PMIOPort  Side=Left
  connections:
  Solid/RConn1 -- ReferenceFrame/RConn1 -- F/RConn1

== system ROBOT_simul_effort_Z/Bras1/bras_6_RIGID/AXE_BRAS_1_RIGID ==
  ReferenceFrame : sm_lib/Frames and Transforms/Reference Frame
  Solid : sm_lib/Body Elements/File Solid  ExtGeomFileName=\STL\AXE BRAS_Defaut_sldprt.STL  UnitType=Custom  ExtGeomFileUnits=mm  StepReaderType=HEX  ExportConvexHullGeometry=off  InertiaType=Custom  Mass=0.0015327306958088996  MassUnits=kg  CenterOfMass=[0 0 0]  CenterOfMassUnits=mm  MomentsOfInertia=[0.11359646260705632 0.11359646260705632 0.0017137152305883286]  MomentsOfInertiaUnits=kg*mm^2  ProductsOfInertia=[0 0 0]  ProductsOfInertiaUnits=kg*mm^2  BasedOnType=Density  Density=1000  DensityUnits=kg/(m^3)  DoExposeReferenceFrame=on  SerializedFrames=<Frames/>  GraphicType=FromGeometry  MarkerShape=Sphere  MarkerSize=10  MarkerSizeUnits=m  GraphicVisPropType=SimpleVisualProperties  GraphicDiffuseColor=[0.6470588235294118 0.61960784313725492 0.58823529411764708]  GraphicSpecularColor=[0.5 0.5 0.5 1.0]  GraphicAmbientColor=[0.15 0.15 0.15 1.0]  GraphicEmissiveColor=[0.0 0.0 0.0 1.0]  GraphicShininess=75  GraphicOpacity=1
  F : PMIOPort  Side=Left
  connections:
  Solid/RConn1 -- ReferenceFrame/RConn1 -- F/RConn1

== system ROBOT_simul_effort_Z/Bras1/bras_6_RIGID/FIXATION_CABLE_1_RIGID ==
  ReferenceFrame : sm_lib/Frames and Transforms/Reference Frame
  Solid : sm_lib/Body Elements/File Solid  ExtGeomFileName=\STL\FIXATION CABLE_Defaut_sldprt.STL  UnitType=Custom  ExtGeomFileUnits=mm  StepReaderType=HEX  ExportConvexHullGeometry=off  InertiaType=Custom  Mass=3.2000000000000007e-06  MassUnits=kg  CenterOfMass=[0 0 0.099999999999999992]  CenterOfMassUnits=mm  MomentsOfInertia=[4.2773333333333348e-06 4.2773333333333331e-06 8.5333333333333352e-06]  MomentsOfInertiaUnits=kg*mm^2  ProductsOfInertia=[0 0 0]  ProductsOfInertiaUnits=kg*mm^2  BasedOnType=Density  Density=1000  DensityUnits=kg/(m^3)  DoExposeReferenceFrame=on  SerializedFrames=<Frames/>  GraphicType=FromGeometry  MarkerShape=Sphere  MarkerSize=10  MarkerSizeUnits=m  GraphicVisPropType=SimpleVisualProperties  GraphicDiffuseColor=[0.25098039215686274 0.25098039215686274 0.25098039215686274]  GraphicSpecularColor=[0.5 0.5 0.5 1.0]  GraphicAmbientColor=[0.15 0.15 0.15 1.0]  GraphicEmissiveColor=[0.0 0.0 0.0 1.0]  GraphicShininess=75  GraphicOpacity=1
  F : PMIOPort  Side=Left
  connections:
  Solid/RConn1 -- ReferenceFrame/RConn1 -- F/RConn1

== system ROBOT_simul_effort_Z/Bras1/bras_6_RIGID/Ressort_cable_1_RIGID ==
  ReferenceFrame : sm_lib/Frames and Transforms/Reference Frame
  Solid : sm_lib/Body Elements/File Solid  ExtGeomFileName=\STL\Ressort cable_Defaut_sldprt.STL  UnitType=Custom  ExtGeomFileUnits=mm  StepReaderType=HEX  ExportConvexHullGeometry=off  InertiaType=Custom  Mass=0.0011765814520035881  MassUnits=kg  CenterOfMass=[0.086849073647483815 -0.00090479521327996976 6.9508776157243597]  CenterOfMassUnits=mm  MomentsOfInertia=[0.034952381374405594 0.034338972761516762 0.0097063586011258158]  MomentsOfInertiaUnits=kg*mm^2  ProductsOfInertia=[0.00037229322226744533 1.6947615167207185e-06 2.0937803976811866e-06]  ProductsOfInertiaUnits=kg*mm^2  BasedOnType=Density  Density=1000  DensityUnits=kg/(m^3)  DoExposeReferenceFrame=on  SerializedFrames=<Frames/>  GraphicType=FromGeometry  MarkerShape=Sphere  MarkerSize=10  MarkerSizeUnits=m  GraphicVisPropType=SimpleVisualProperties  GraphicDiffuseColor=[0.0 0.0 0.0]  GraphicSpecularColor=[0.5 0.5 0.5 1.0]  GraphicAmbientColor=[0.15 0.15 0.15 1.0]  GraphicEmissiveColor=[0.0 0.0 0.0 1.0]  GraphicShininess=75  GraphicOpacity=1
  F : PMIOPort  Side=Left
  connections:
  Solid/RConn1 -- ReferenceFrame/RConn1 -- F/RConn1

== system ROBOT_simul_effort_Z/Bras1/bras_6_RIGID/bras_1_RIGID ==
  ReferenceFrame : sm_lib/Frames and Transforms/Reference Frame
  Solid : sm_lib/Body Elements/File Solid  ExtGeomFileName=\STL\bras_Defaut_sldprt.STL  UnitType=Custom  ExtGeomFileUnits=mm  StepReaderType=HEX  ExportConvexHullGeometry=off  InertiaType=Custom  Mass=0.06566875822643542  MassUnits=kg  CenterOfMass=[23.925748169887701 -4.7774352723885904 0.0071346362933715022]  CenterOfMassUnits=mm  MomentsOfInertia=[75.153076467382206 23.577652078949701 94.231108050856861]  MomentsOfInertiaUnits=kg*mm^2  ProductsOfInertia=[0.01532312637695204 0.0017211125494294708 -5.8798668472039237]  ProductsOfInertiaUnits=kg*mm^2  BasedOnType=Density  Density=1000  DensityUnits=kg/(m^3)  DoExposeReferenceFrame=on  SerializedFrames=<Frames/>  GraphicType=FromGeometry  MarkerShape=Sphere  MarkerSize=10  MarkerSizeUnits=m  GraphicVisPropType=SimpleVisualProperties  GraphicDiffuseColor=[1.0 1.0 0.0]  GraphicSpecularColor=[0.5 0.5 0.5 1.0]  GraphicAmbientColor=[0.15 0.15 0.15 1.0]  GraphicEmissiveColor=[0.0 0.0 0.0 1.0]  GraphicShininess=75  GraphicOpacity=1
  F : PMIOPort  Side=Left
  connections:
  Solid/RConn1 -- ReferenceFrame/RConn1 -- F/RConn1

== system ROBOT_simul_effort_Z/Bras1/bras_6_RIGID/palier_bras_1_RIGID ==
  ReferenceFrame : sm_lib/Frames and Transforms/Reference Frame
  Solid : sm_lib/Body Elements/File Solid  ExtGeomFileName=\STL\palier bras_Defaut_sldprt.STL  UnitType=Custom  ExtGeomFileUnits=mm  StepReaderType=HEX  ExportConvexHullGeometry=off  InertiaType=Custom  Mass=0.00017920168094851793  MassUnits=kg  CenterOfMass=[-178.32667601154176 39.825618202078154 -20.980989744703667]  CenterOfMassUnits=mm  MomentsOfInertia=[0.0018602253674838991 0.0012789874237151958 0.0012789874237151961]  MomentsOfInertiaUnits=kg*mm^2  ProductsOfInertia=[0 0 0]  ProductsOfInertiaUnits=kg*mm^2  BasedOnType=Density  Density=1000  DensityUnits=kg/(m^3)  DoExposeReferenceFrame=on  SerializedFrames=<Frames/>  GraphicType=FromGeometry  MarkerShape=Sphere  MarkerSize=10  MarkerSizeUnits=m  GraphicVisPropType=SimpleVisualProperties  GraphicDiffuseColor=[1 1 1]  GraphicSpecularColor=[0.5 0.5 0.5 1.0]  GraphicAmbientColor=[0.15 0.15 0.15 1.0]  GraphicEmissiveColor=[0.0 0.0 0.0 1.0]  GraphicShininess=75  GraphicOpacity=1
  F : PMIOPort  Side=Left
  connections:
  Solid/RConn1 -- ReferenceFrame/RConn1 -- F/RConn1

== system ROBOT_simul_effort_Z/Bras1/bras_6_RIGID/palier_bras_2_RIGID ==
  ReferenceFrame : sm_lib/Frames and Transforms/Reference Frame
  Solid : sm_lib/Body Elements/File Solid  ExtGeomFileName=\STL\palier bras_Defaut_sldprt.STL  UnitType=Custom  ExtGeomFileUnits=mm  StepReaderType=HEX  ExportConvexHullGeometry=off  InertiaType=Custom  Mass=0.00017920168094851793  MassUnits=kg  CenterOfMass=[-178.32667601154176 39.825618202078154 -20.980989744703667]  CenterOfMassUnits=mm  MomentsOfInertia=[0.0018602253674838991 0.0012789874237151958 0.0012789874237151961]  MomentsOfInertiaUnits=kg*mm^2  ProductsOfInertia=[0 0 0]  ProductsOfInertiaUnits=kg*mm^2  BasedOnType=Density  Density=1000  DensityUnits=kg/(m^3)  DoExposeReferenceFrame=on  SerializedFrames=<Frames/>  GraphicType=FromGeometry  MarkerShape=Sphere  MarkerSize=10  MarkerSizeUnits=m  GraphicVisPropType=SimpleVisualProperties  GraphicDiffuseColor=[1 1 1]  GraphicSpecularColor=[0.5 0.5 0.5 1.0]  GraphicAmbientColor=[0.15 0.15 0.15 1.0]  GraphicEmissiveColor=[0.0 0.0 0.0 1.0]  GraphicShininess=75  GraphicOpacity=1
  F : PMIOPort  Side=Left
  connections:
  Solid/RConn1 -- ReferenceFrame/RConn1 -- F/RConn1

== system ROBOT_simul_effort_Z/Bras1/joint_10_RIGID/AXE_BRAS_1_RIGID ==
  ReferenceFrame : sm_lib/Frames and Transforms/Reference Frame
  Solid : sm_lib/Body Elements/File Solid  ExtGeomFileName=\STL\AXE BRAS_Defaut_sldprt.STL  UnitType=Custom  ExtGeomFileUnits=mm  StepReaderType=HEX  ExportConvexHullGeometry=off  InertiaType=Custom  Mass=0.0015327306958088996  MassUnits=kg  CenterOfMass=[0 0 0]  CenterOfMassUnits=mm  MomentsOfInertia=[0.11359646260705632 0.11359646260705632 0.0017137152305883286]  MomentsOfInertiaUnits=kg*mm^2  ProductsOfInertia=[0 0 0]  ProductsOfInertiaUnits=kg*mm^2  BasedOnType=Density  Density=1000  DensityUnits=kg/(m^3)  DoExposeReferenceFrame=on  SerializedFrames=<Frames/>  GraphicType=FromGeometry  MarkerShape=Sphere  MarkerSize=10  MarkerSizeUnits=m  GraphicVisPropType=SimpleVisualProperties  GraphicDiffuseColor=[0.6470588235294118 0.61960784313725492 0.58823529411764708]  GraphicSpecularColor=[0.5 0.5 0.5 1.0]  GraphicAmbientColor=[0.15 0.15 0.15 1.0]  GraphicEmissiveColor=[0.0 0.0 0.0 1.0]  GraphicShininess=75  GraphicOpacity=1
  F : PMIOPort  Side=Left
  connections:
  Solid/RConn1 -- ReferenceFrame/RConn1 -- F/RConn1

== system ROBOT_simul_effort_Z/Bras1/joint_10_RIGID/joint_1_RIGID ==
  ReferenceFrame : sm_lib/Frames and Transforms/Reference Frame
  Solid : sm_lib/Body Elements/File Solid  ExtGeomFileName=\STL\joint_Defaut_sldprt.STL  UnitType=Custom  ExtGeomFileUnits=mm  StepReaderType=HEX  ExportConvexHullGeometry=off  InertiaType=Custom  Mass=0.0062454336323428689  MassUnits=kg  CenterOfMass=[-4.7519597301086606e-06 14.873568128586268 0.2827021501004604]  CenterOfMassUnits=mm  MomentsOfInertia=[0.43544209184236687 0.81590742360241675 0.91424830357082487]  MomentsOfInertiaUnits=kg*mm^2  ProductsOfInertia=[0.0068320776316595647 -4.173068650825101e-06 -7.5142319098046527e-07]  ProductsOfInertiaUnits=kg*mm^2  BasedOnType=Density  Density=1000  DensityUnits=kg/(m^3)  DoExposeReferenceFrame=on  SerializedFrames=<Frames/>  GraphicType=FromGeometry  MarkerShape=Sphere  MarkerSize=10  MarkerSizeUnits=m  GraphicVisPropType=SimpleVisualProperties  GraphicDiffuseColor=[1 1 1]  GraphicSpecularColor=[0.5 0.5 0.5 1.0]  GraphicAmbientColor=[0.15 0.15 0.15 1.0]  GraphicEmissiveColor=[0.0 0.0 0.0 1.0]  GraphicShininess=75  GraphicOpacity=1
  F : PMIOPort  Side=Left
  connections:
  Solid/RConn1 -- ReferenceFrame/RConn1 -- F/RConn1

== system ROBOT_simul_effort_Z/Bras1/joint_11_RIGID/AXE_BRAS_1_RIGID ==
  ReferenceFrame : sm_lib/Frames and Transforms/Reference Frame
  Solid : sm_lib/Body Elements/File Solid  ExtGeomFileName=\STL\AXE BRAS_Defaut_sldprt.STL  UnitType=Custom  ExtGeomFileUnits=mm  StepReaderType=HEX  ExportConvexHullGeometry=off  InertiaType=Custom  Mass=0.0015327306958088996  MassUnits=kg  CenterOfMass=[0 0 0]  CenterOfMassUnits=mm  MomentsOfInertia=[0.11359646260705632 0.11359646260705632 0.0017137152305883286]  MomentsOfInertiaUnits=kg*mm^2  ProductsOfInertia=[0 0 0]  ProductsOfInertiaUnits=kg*mm^2  BasedOnType=Density  Density=1000  DensityUnits=kg/(m^3)  DoExposeReferenceFrame=on  SerializedFrames=<Frames/>  GraphicType=FromGeometry  MarkerShape=Sphere  MarkerSize=10  MarkerSizeUnits=m  GraphicVisPropType=SimpleVisualProperties  GraphicDiffuseColor=[0.6470588235294118 0.61960784313725492 0.58823529411764708]  GraphicSpecularColor=[0.5 0.5 0.5 1.0]  GraphicAmbientColor=[0.15 0.15 0.15 1.0]  GraphicEmissiveColor=[0.0 0.0 0.0 1.0]  GraphicShininess=75  GraphicOpacity=1
  F : PMIOPort  Side=Left
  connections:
  Solid/RConn1 -- ReferenceFrame/RConn1 -- F/RConn1

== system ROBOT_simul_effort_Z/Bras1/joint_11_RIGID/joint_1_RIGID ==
  ReferenceFrame : sm_lib/Frames and Transforms/Reference Frame
  Solid : sm_lib/Body Elements/File Solid  ExtGeomFileName=\STL\joint_Defaut_sldprt.STL  UnitType=Custom  ExtGeomFileUnits=mm  StepReaderType=HEX  ExportConvexHullGeometry=off  InertiaType=Custom  Mass=0.0062454336323428689  MassUnits=kg  CenterOfMass=[-4.7519597301086606e-06 14.873568128586268 0.2827021501004604]  CenterOfMassUnits=mm  MomentsOfInertia=[0.43544209184236687 0.81590742360241675 0.91424830357082487]  MomentsOfInertiaUnits=kg*mm^2  ProductsOfInertia=[0.0068320776316595647 -4.173068650825101e-06 -7.5142319098046527e-07]  ProductsOfInertiaUnits=kg*mm^2  BasedOnType=Density  Density=1000  DensityUnits=kg/(m^3)  DoExposeReferenceFrame=on  SerializedFrames=<Frames/>  GraphicType=FromGeometry  MarkerShape=Sphere  MarkerSize=10  MarkerSizeUnits=m  GraphicVisPropType=SimpleVisualProperties  GraphicDiffuseColor=[1 1 1]  GraphicSpecularColor=[0.5 0.5 0.5 1.0]  GraphicAmbientColor=[0.15 0.15 0.15 1.0]  GraphicEmissiveColor=[0.0 0.0 0.0 1.0]  GraphicShininess=75  GraphicOpacity=1
  F : PMIOPort  Side=Left
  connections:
  Solid/RConn1 -- ReferenceFrame/RConn1 -- F/RConn1

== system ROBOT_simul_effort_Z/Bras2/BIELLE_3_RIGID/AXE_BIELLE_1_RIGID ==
  ReferenceFrame : sm_lib/Frames and Transforms/Reference Frame
  Solid : sm_lib/Body Elements/File Solid  ExtGeomFileName=\STL\AXE BIELLE_Defaut_sldprt.STL  UnitType=Custom  ExtGeomFileUnits=mm  StepReaderType=HEX  ExportConvexHullGeometry=off  InertiaType=Custom  Mass=0.0008880235381781051  MassUnits=kg  CenterOfMass=[0 0 0]  CenterOfMassUnits=mm  MomentsOfInertia=[0.018768660222737772 0.018768660222737772 0.0009874025874388381]  MomentsOfInertiaUnits=kg*mm^2  ProductsOfInertia=[0 0 0]  ProductsOfInertiaUnits=kg*mm^2  BasedOnType=Density  Density=1000  DensityUnits=kg/(m^3)  DoExposeReferenceFrame=on  SerializedFrames=<Frames/>  GraphicType=FromGeometry  MarkerShape=Sphere  MarkerSize=10  MarkerSizeUnits=m  GraphicVisPropType=SimpleVisualProperties  GraphicDiffuseColor=[1 0.94901960784313721 0.90980392156862744]  GraphicSpecularColor=[0.5 0.5 0.5 1.0]  GraphicAmbientColor=[0.15 0.15 0.15 1.0]  GraphicEmissiveColor=[0.0 0.0 0.0 1.0]  GraphicShininess=75  GraphicOpacity=1
  F : PMIOPort  Side=Left
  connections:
  Solid/RConn1 -- ReferenceFrame/RConn1 -- F/RConn1

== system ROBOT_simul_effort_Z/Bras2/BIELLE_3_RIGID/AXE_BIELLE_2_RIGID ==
  ReferenceFrame : sm_lib/Frames and Transforms/Reference Frame
  Solid : sm_lib/Body Elements/File Solid  ExtGeomFileName=\STL\AXE BIELLE_Defaut_sldprt.STL  UnitType=Custom  ExtGeomFileUnits=mm  StepReaderType=HEX  ExportConvexHullGeometry=off  InertiaType=Custom  Mass=0.0008880235381781051  MassUnits=kg  CenterOfMass=[0 0 0]  CenterOfMassUnits=mm  MomentsOfInertia=[0.018768660222737772 0.018768660222737772 0.0009874025874388381]  MomentsOfInertiaUnits=kg*mm^2  ProductsOfInertia=[0 0 0]  ProductsOfInertiaUnits=kg*mm^2  BasedOnType=Density  Density=1000  DensityUnits=kg/(m^3)  DoExposeReferenceFrame=on  SerializedFrames=<Frames/>  GraphicType=FromGeometry  MarkerShape=Sphere  MarkerSize=10  MarkerSizeUnits=m  GraphicVisPropType=SimpleVisualProperties  GraphicDiffuseColor=[1 0.94901960784313721 0.90980392156862744]  GraphicSpecularColor=[0.5 0.5 0.5 1.0]  GraphicAmbientColor=[0.15 0.15 0.15 1.0]  GraphicEmissiveColor=[0.0 0.0 0.0 1.0]  GraphicShininess=75  GraphicOpacity=1
  F : PMIOPort  Side=Left
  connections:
  Solid/RConn1 -- ReferenceFrame/RConn1 -- F/RConn1

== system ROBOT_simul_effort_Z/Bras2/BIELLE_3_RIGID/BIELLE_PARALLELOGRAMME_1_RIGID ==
  ReferenceFrame : sm_lib/Frames and Transforms/Reference Frame
  Solid : sm_lib/Body Elements/File Solid  ExtGeomFileName=\STL\BIELLE PARALLELOGRAMME_Defaut_sldprt.STL  UnitType=Custom  ExtGeomFileUnits=mm  StepReaderType=HEX  ExportConvexHullGeometry=off  InertiaType=Custom  Mass=0.0079529027635324764  MassUnits=kg  CenterOfMass=[0 3.1653377955585489 0]  CenterOfMassUnits=mm  MomentsOfInertia=[7.7987017961340088 7.8475939194203406 0.14816857834406802]  MomentsOfInertiaUnits=kg*mm^2  ProductsOfInertia=[0 0 0]  ProductsOfInertiaUnits=kg*mm^2  BasedOnType=Density  Density=1000  DensityUnits=kg/(m^3)  DoExposeReferenceFrame=on  SerializedFrames=<Frames/>  GraphicType=FromGeometry  MarkerShape=Sphere  MarkerSize=10  MarkerSizeUnits=m  GraphicVisPropType=SimpleVisualProperties  GraphicDiffuseColor=[0.6 1.0 1.0]  GraphicSpecularColor=[0.5 0.5 0.5 1.0]  GraphicAmbientColor=[0.15 0.15 0.15 1.0]  GraphicEmissiveColor=[0.0 0.0 0.0 1.0]  GraphicShininess=75  GraphicOpacity=1
  F : PMIOPort  Side=Left
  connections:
  Solid/RConn1 -- ReferenceFrame/RConn1 -- F/RConn1

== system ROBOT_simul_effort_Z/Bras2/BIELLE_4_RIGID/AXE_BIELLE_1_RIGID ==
  ReferenceFrame : sm_lib/Frames and Transforms/Reference Frame
  Solid : sm_lib/Body Elements/File Solid  ExtGeomFileName=\STL\AXE BIELLE_Defaut_sldprt.STL  UnitType=Custom  ExtGeomFileUnits=mm  StepReaderType=HEX  ExportConvexHullGeometry=off  InertiaType=Custom  Mass=0.0008880235381781051  MassUnits=kg  CenterOfMass=[0 0 0]  CenterOfMassUnits=mm  MomentsOfInertia=[0.018768660222737772 0.018768660222737772 0.0009874025874388381]  MomentsOfInertiaUnits=kg*mm^2  ProductsOfInertia=[0 0 0]  ProductsOfInertiaUnits=kg*mm^2  BasedOnType=Density  Density=1000  DensityUnits=kg/(m^3)  DoExposeReferenceFrame=on  SerializedFrames=<Frames/>  GraphicType=FromGeometry  MarkerShape=Sphere  MarkerSize=10  MarkerSizeUnits=m  GraphicVisPropType=SimpleVisualProperties  GraphicDiffuseColor=[1 0.94901960784313721 0.90980392156862744]  GraphicSpecularColor=[0.5 0.5 0.5 1.0]  GraphicAmbientColor=[0.15 0.15 0.15 1.0]  GraphicEmissiveColor=[0.0 0.0 0.0 1.0]  GraphicShininess=75  GraphicOpacity=1
  F : PMIOPort  Side=Left
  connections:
  Solid/RConn1 -- ReferenceFrame/RConn1 -- F/RConn1

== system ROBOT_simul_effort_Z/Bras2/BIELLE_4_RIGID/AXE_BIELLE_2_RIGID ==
  ReferenceFrame : sm_lib/Frames and Transforms/Reference Frame
  Solid : sm_lib/Body Elements/File Solid  ExtGeomFileName=\STL\AXE BIELLE_Defaut_sldprt.STL  UnitType=Custom  ExtGeomFileUnits=mm  StepReaderType=HEX  ExportConvexHullGeometry=off  InertiaType=Custom  Mass=0.0008880235381781051  MassUnits=kg  CenterOfMass=[0 0 0]  CenterOfMassUnits=mm  MomentsOfInertia=[0.018768660222737772 0.018768660222737772 0.0009874025874388381]  MomentsOfInertiaUnits=kg*mm^2  ProductsOfInertia=[0 0 0]  ProductsOfInertiaUnits=kg*mm^2  BasedOnType=Density  Density=1000  DensityUnits=kg/(m^3)  DoExposeReferenceFrame=on  SerializedFrames=<Frames/>  GraphicType=FromGeometry  MarkerShape=Sphere  MarkerSize=10  MarkerSizeUnits=m  GraphicVisPropType=SimpleVisualProperties  GraphicDiffuseColor=[1 0.94901960784313721 0.90980392156862744]  GraphicSpecularColor=[0.5 0.5 0.5 1.0]  GraphicAmbientColor=[0.15 0.15 0.15 1.0]  GraphicEmissiveColor=[0.0 0.0 0.0 1.0]  GraphicShininess=75  GraphicOpacity=1
  F : PMIOPort  Side=Left
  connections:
  Solid/RConn1 -- ReferenceFrame/RConn1 -- F/RConn1
